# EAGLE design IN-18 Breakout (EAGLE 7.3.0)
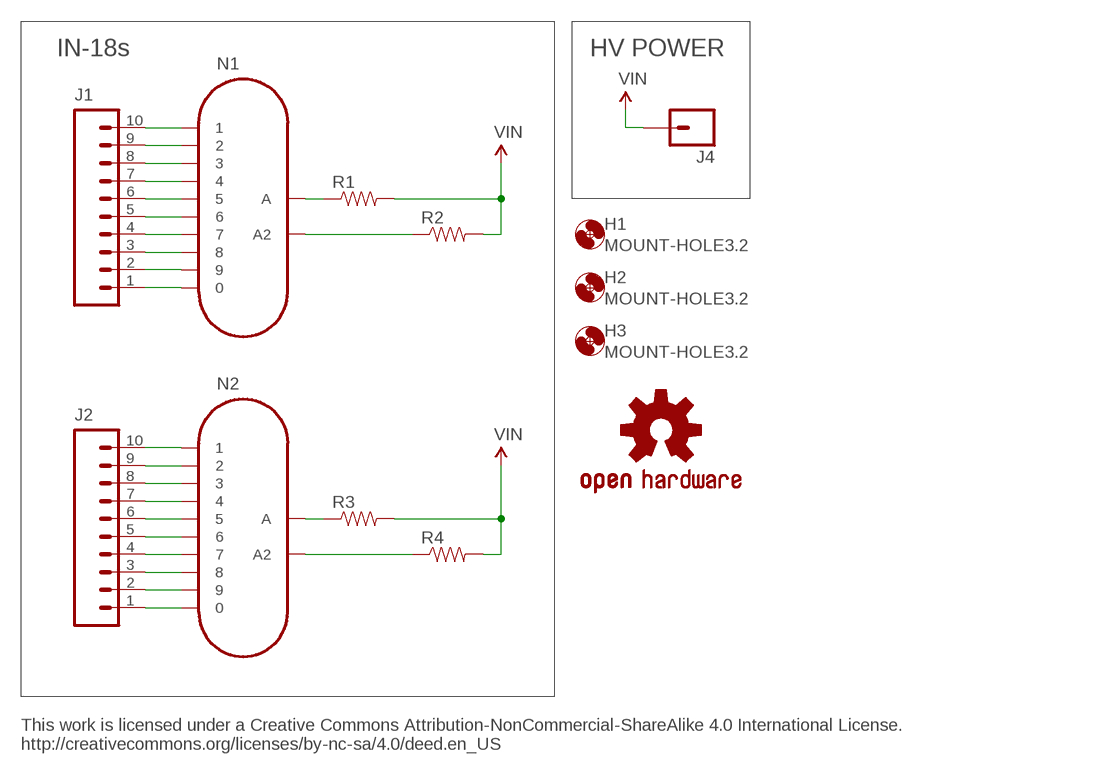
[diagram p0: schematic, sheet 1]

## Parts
H1  MOUNT-HOLE3.2  [3,2]
H2  MOUNT-HOLE3.2  [3,2]
H3  MOUNT-HOLE3.2  [3,2]
J1  M10SILK_FEMALE_PTH  [1X10]
J2  M10SILK_FEMALE_PTH  [1X10]
J4  M01PTH_LONGPAD  [1X01_LONGPAD]
N1  IN-18  [IN-18]
N2  IN-18  [IN-18]
R1  RESISTORPTH-1/4W  [AXIAL-0.4]
R2  RESISTORPTH-1/4W  [AXIAL-0.4]
R3  RESISTORPTH-1/4W  [AXIAL-0.4]
R4  RESISTORPTH-1/4W  [AXIAL-0.4]
U$4  OSHW-LOGOM  [OSHW-LOGO-M]

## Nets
N$1: J1.10 N1.1
N$2: N1.A R1.P$1
N$3: J1.9 N1.2
N$4: J1.8 N1.3
N$5: J1.7 N1.4
N$6: N2.A2 R4.P$1
N$7: J1.6 N1.5
N$12: J1.5 N1.6
N$16: J1.4 N1.7
N$17: J1.3 N1.8
N$18: J1.2 N1.9
N$19: J1.1 N1.0
N$20: J2.10 N2.1
N$21: J2.9 N2.2
N$22: J2.8 N2.3
N$23: J2.7 N2.4
N$24: J2.6 N2.5
N$25: J2.5 N2.6
N$26: J2.4 N2.7
N$27: J2.3 N2.8
N$28: J2.2 N2.9
N$29: J2.1 N2.0
N$30: N2.A R3.P$1
N$42: N1.A2 R2.P$1
VIN: J4.1 R1.P$2 R2.P$2 R3.P$2 R4.P$2

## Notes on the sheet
- IN-18s | HV POWER
- This work is licensed under a Creative Commons Attribution-NonCommercial-ShareAlike 4.0 International License.
  http://creativecommons.org/licenses/by-nc-sa/4.0/deed.en_US

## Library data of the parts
H1-H3 = holes:MOUNT-HOLE: MOUNTING HOLE with drill center marker
J1 J2 = SparkFun-Connectors:M10: Header 10 Standard 10-pin 0.1" header. Use with straight break away headers (SKU : PRT-00116), right angle break away headers (PRT-00553), swiss pins (PRT-00743), machine pins (PRT-00117), and female headers (PRT-00115).; PROD_ID: CONN-11563
J4 = SparkFun-Connectors:M01: Header 1
N1 N2 = Nixie Tubes 2:IN-18: IN-18: large numeric frontview nixie tube
R1-R4 = SparkFun-Resistors:RESISTOR: Resistor
U$4 = SparkFun:OSHW-LOGO: Open Source Hardware Logo This logo indicates the piece of hardware it is found on incorporates a OSHW license and/or adheres to the definition of open source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

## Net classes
0 default: width 0.254 mm

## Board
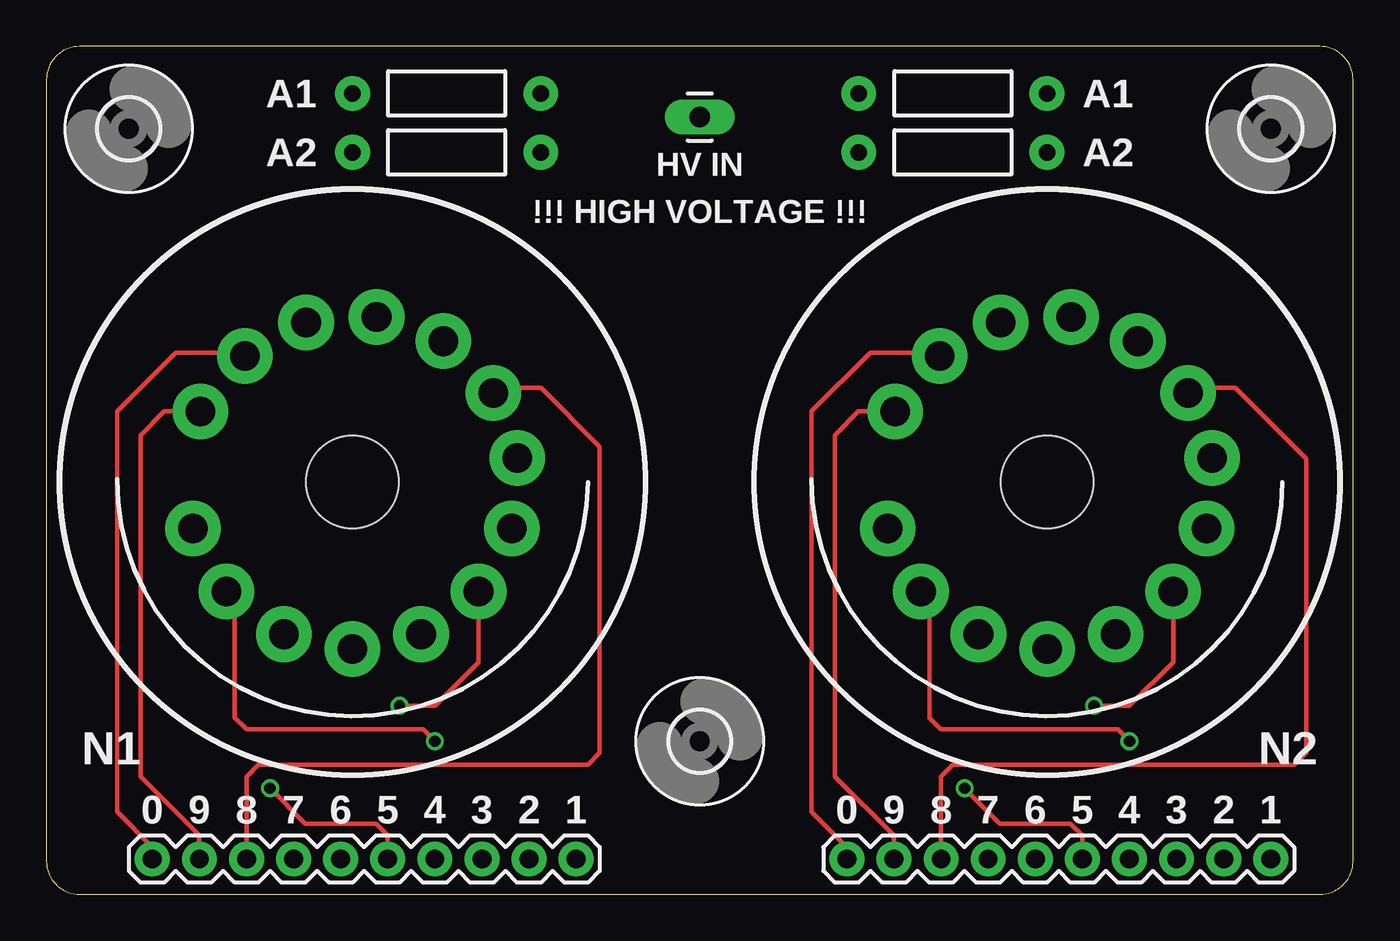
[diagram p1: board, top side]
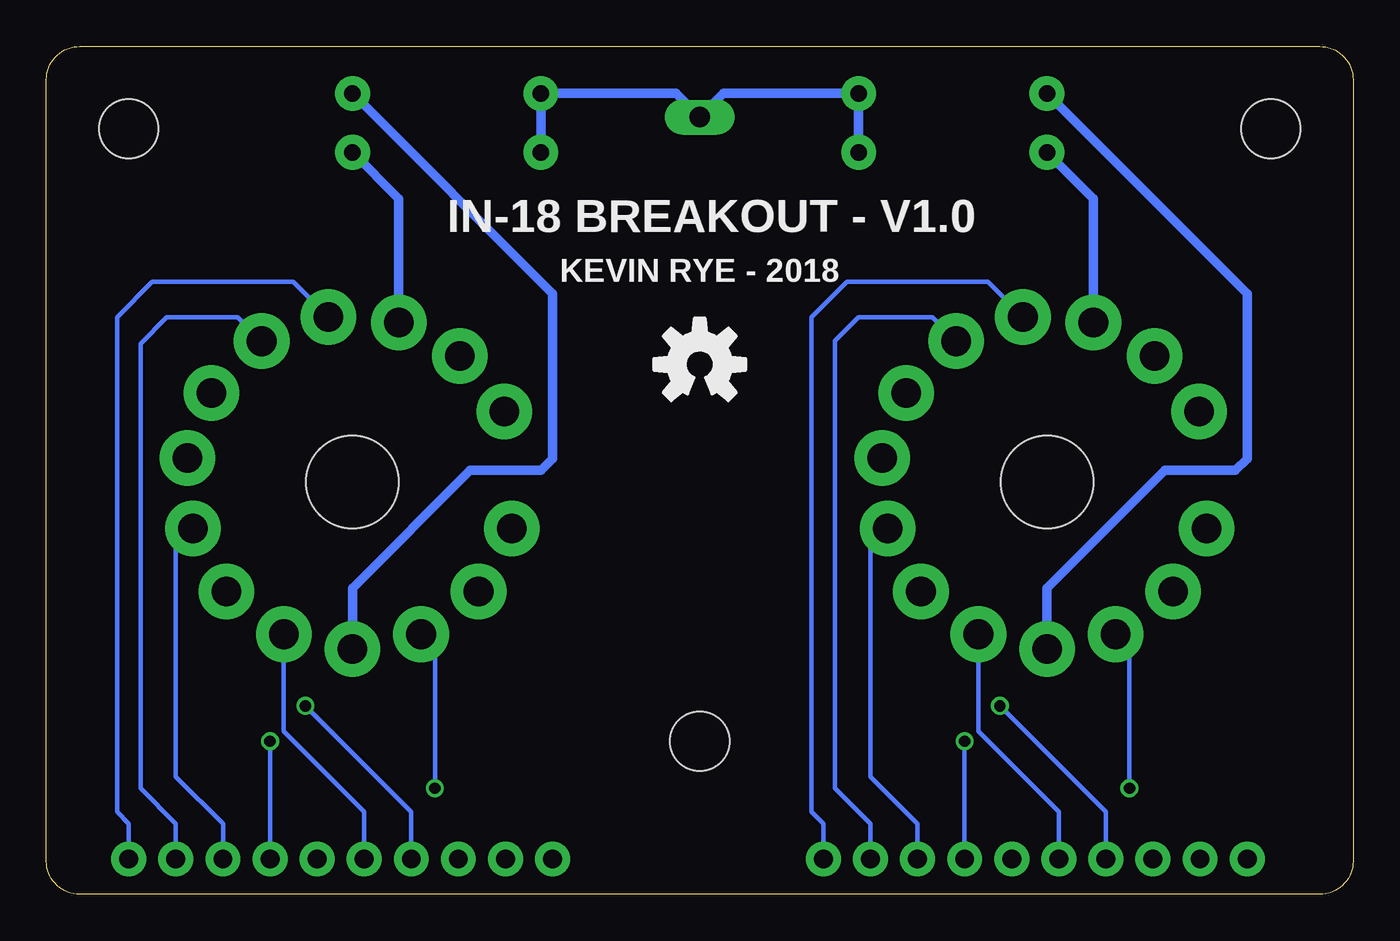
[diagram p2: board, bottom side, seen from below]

Size 70.48 x 45.72 mm. Coordinates in mm from the lower left corner, seen from the top.
Outline: 0,43.92 0,1.8 arc90 1.8,0 68.69,0 arc90 70.48,1.8 70.48,43.92 arc90 68.69,45.72 1.8,45.72 arc90 0,43.92
Copper layers (1*16): Top 0.0356mm / dielectric 1.5011mm / Bottom 0.0356mm
Design rules "oshpark-2layer": minimum track width 6mil, minimum drill 13mil, track to track 6mil, track to pad 6mil, pad to pad 6mil, via to via 6mil, smd to smd 6mil, copper to edge 15mil, drill to drill 6mil, minimum pad ring 7mil, minimum via ring 7mil, stop-mask expansion 2.5mil, vias tented up to drill 0mil, thermal gap 10mil

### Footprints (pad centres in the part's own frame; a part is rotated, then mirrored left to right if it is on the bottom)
3,2 = hole 3.2: 0,0
1X10 = drill 1.016 pad 1.88: 1 0,0; 2 2.54,0; 3 5.08,0; 4 7.62,0; 5 10.16,0; 6 12.7,0; 7 15.24,0; 8 17.78,0; 9 20.32,0; 10 22.86,0
1X01_LONGPAD = drill 1.118 pad 1.88 long: 1 0,0
IN-18 = drill 1.6 pad 3: 0 5.8,-6.8; 1 -1.3,-8.9; 2 -4.9,-7.6; 3 -8.6,2.5; 4 6.8,5.9; 5 3.7,8.2; 6 -3.7,8.2; 7 -6.8,5.9; 8 -7.6,-4.8; 9 8.2,-3.8; A 0,9; A2 2.5,-8.6; N/C 8.6,2.5; N/C2 -8.9,-1.3 | hole 5: 0,0
AXIAL-0.4 = drill 0.9 pad 1.88: P$1 -5.08,0; P$2 5.08,0

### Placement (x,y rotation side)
H1  66.04,41.27 0 top
H2  4.45,41.27 0 top
H3  35.24,8.25 0 top
J1  5.71,1.91 0 top
J2  43.18,1.91 0 top
J4  35.24,41.91 90 top
N1  16.51,22.23 180 top
N2  53.98,22.23 180 top
R1  21.59,43.18 0 top
R2  21.59,40.01 0 top
R3  48.9,43.18 180 top
R4  48.9,40.01 180 top
U$4  35.24,28.57 0 bottom

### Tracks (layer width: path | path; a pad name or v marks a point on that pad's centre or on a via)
N$1
  Bottom 0.254: N1.1 19.7,33.02 27.3,33.02 29.21,31.12 29.21,4.45 28.57,3.81 J1.10
N$2
  Bottom 0.508: R1.P$1 5.71,32.38 5.71,23.5 6.35,22.86 10.16,22.86 16.51,16.51 N1.A
N$3
  Bottom 0.254: N1.2 22.7,31.12 26.67,31.12 27.94,29.84 27.94,5.72 26.04,3.81 J1.9
N$4
  Bottom 0.254: J1.8 23.5,3.81 26.04,6.35 26.04,18.8 N1.3
N$5  (via drill 0.61)
  Top 0.254: N1.4 10.16,15.88 10.16,9.52 10.79,8.89 20.32,8.89 v20.95,8.25
  Bottom 0.254: v20.95,8.25 J1.7
N$6
  Bottom 0.508: R4.P$1 51.48,37.51 N2.A2
N$7  (via drill 0.61)
  Top 0.254: v12.06,5.72 13.97,3.81 17.78,3.81 18.41,3.17 J1.6
  Bottom 0.254: N1.5 12.06,13.28 v12.06,5.72
N$12
  Bottom 0.254: J1.5 15.88,4.45 20.21,8.78 N1.6
N$16  (via drill 0.61)
  Top 0.254: v19.05,10.16 20.95,10.16 23.31,12.52 N1.7
  Bottom 0.254: J1.4 13.34,4.45 v19.05,10.16
N$17
  Top 0.254: J1.3 10.79,6.35 11.43,6.99 29.21,6.99 29.84,7.62 29.84,24.13 26.67,27.3 24.39,27.3 N1.8
N$18
  Top 0.254: J1.2 8.26,3.17 5.08,6.35 5.08,24.77 6.35,26.04 N1.9
N$19
  Top 0.254: J1.1 5.71,2.54 3.81,4.45 3.81,26.04 6.99,29.21 10.53,29.21 N1.0
N$20
  Bottom 0.254: N2.1 57.17,33.02 64.77,33.02 66.67,31.12 66.67,4.45 66.04,3.81 J2.10
N$21
  Bottom 0.254: N2.2 60.16,31.12 63.98,31.12 65.41,29.7 65.41,5.72 63.5,3.81 J2.9
N$22
  Bottom 0.254: J2.8 60.96,3.81 63.5,6.35 63.5,18.8 N2.3
N$23  (via drill 0.61)
  Top 0.254: N2.4 47.62,15.88 47.62,9.52 48.26,8.89 57.78,8.89 v58.42,8.25
  Bottom 0.254: v58.42,8.25 J2.7
N$24  (via drill 0.61)
  Top 0.254: v49.53,5.72 51.44,3.81 55.24,3.81 55.88,3.17 J2.6
  Bottom 0.254: N2.5 49.53,13.28 v49.53,5.72
N$25
  Bottom 0.254: J2.5 53.34,4.45 57.67,8.78 N2.6
N$26  (via drill 0.61)
  Top 0.254: v56.52,10.16 58.42,10.16 60.77,12.52 N2.7
  Bottom 0.254: J2.4 50.8,4.45 v56.52,10.16
N$27
  Top 0.254: J2.3 48.26,6.35 48.9,6.99 67.31,6.99 67.94,7.62 67.94,23.5 64.14,27.3 61.85,27.3 N2.8
N$28
  Top 0.254: J2.2 45.72,3.17 42.55,6.35 42.55,24.77 43.81,26.04 45.77,26.04 N2.9
N$29
  Top 0.254: J2.1 43.18,2.54 41.27,4.45 41.27,26.04 44.45,29.21 47.99,29.21 N2.0
N$30
  Bottom 0.508: R3.P$1 43.18,32.38 43.18,23.5 43.81,22.86 47.62,22.86 53.98,16.51 N2.A
N$42
  Bottom 0.508: R2.P$1 14.01,37.51 N1.A2
VIN
  Bottom 0.508: R4.P$2 R3.P$2 36.51,43.18 J4.1 33.97,43.18 R1.P$2 R2.P$2

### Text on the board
Unrouted: This work is licensed under a Creative Commons Attribution-NonCommercial-ShareAlike 4.0 International License. / http://creativecommons.org/licenses/by-nc-sa/4.0/deed.en_US
tNames: A1 | A1 | A2 | HV IN | A2 | !!! HIGH VOLTAGE !!! | N1 | N2 | 0 | 9 | 8 | 7 | 6 | 5 | 4 | 3 | 2 | 1 | 0 | 9 | 8 | 7 | 6 | 5 | 4 | 3 | 2 | 1
bNames: IN-18 BREAKOUT - V1.0 | KEVIN RYE - 2018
